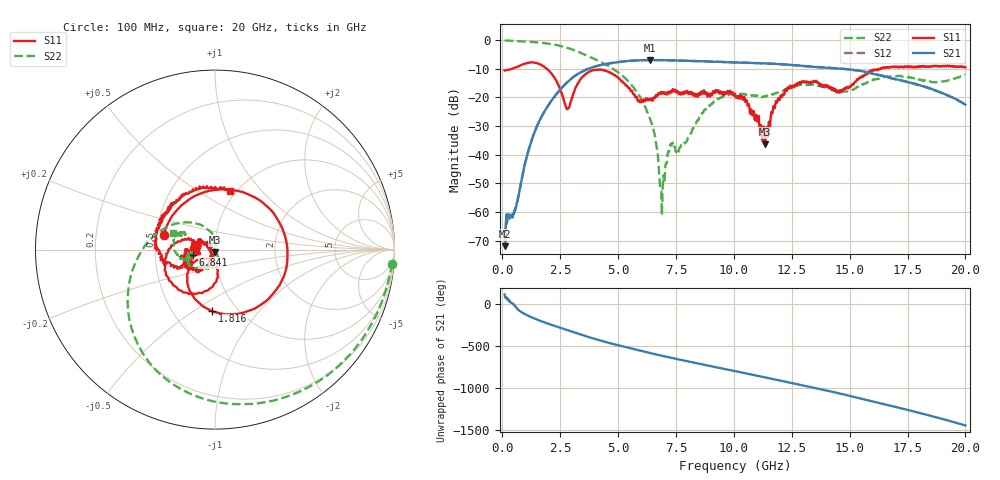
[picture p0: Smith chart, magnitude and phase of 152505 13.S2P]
!  2-Port S-parameters saved by WinCal
! VAR MeasName=S-Parameters (CALIBRATED_DATA) read from VNA (N5230C)
! VAR MeasDate=4/10/2015 9:29:35 AM
! VAR NAME=152505 13
! VAR FILENAME=152505 13.S2P
! VAR DATE=4/10/2015 9:29:35 AM
! VAR PHYS_PORTS=1,2
# Hz S DB R 50
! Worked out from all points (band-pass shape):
!   801 points, 100 MHz to 20 GHz, reference 50 ohm
!   highest |S21| = -6.92 dB at 6.393 GHz (marker M1); lowest = -71.9 dB at 124.9 MHz (marker M2)
!   |S21| within 3 dB of the highest: 3.733 GHz to 14.57 GHz (10.84 GHz wide, 118 % of centre)
!   lowest |S11| = -36.4 dB at 11.34 GHz (marker M3), VSWR 1.03, Z = 49.8 - j1.51 ohm
!   |S11| at or under -10 dB: start of sweep to 413.4 MHz; 1.927 GHz to 16.32 GHz (14.39 GHz wide, 158 % of centre)
!   |S22| runs from -61.1 to -0.1 dB; largest |S21 - S12| = 0.0063
!   S11 on the Smith chart (normalised r, x): 100 MHz: 0.55, +0.10; 1.816 GHz: 0.77, -0.60; 6.841 GHz: 0.78, -0.05; 20 GHz: 0.94, +0.69
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1e8  -10.57 164.5  -67.38 110.1  -70.23 114.6  -0.08 -4.6
1.24875e8  -10.54 160.5  -71.92 74.5  -68.42 97.4  -0.10 -5.5
6.4725e8  -9.29 77.1  -56.43 -58.5  -56.48 -58.9  -0.31 -26.3
1.095e9  -7.94 5.0  -39.47 -139.7  -39.52 -139.5  -0.50 -44.3
1.816375e9  -9.27 -92.6  -24.94 138.8  -24.94 138.9  -1.02 -74.2
2.811375e9  -23.99 -118.8  -14.63 46.1  -14.64 46.4  -2.65 -118.3
3.43325e9  -13.11 -98.1  -11.03 -10.9  -11.00 -10.6  -4.56 -145.0
4.701875e9  -11.53 -175.9  -8.02 -112.6  -8.00 -112.4  -9.54 163.8
5.5725e9  -17.67 156.1  -7.16 -173.5  -7.14 -173.7  -15.50 122.3
6.393375e9  -20.97 -167.2  -6.92 132.3  -6.93 132.3  -27.70 85.4
6.741625e9  -18.51 -168.6  -6.95 110.5  -6.93 110.2  -42.78 82.0
6.841125e9  -18.04 -166.6  -6.95 104.3  -6.97 104.0  -52.24 142.4
7.264e9  -17.75 -173.8  -7.04 78.8  -7.03 78.8  -36.29 -130.2
8.582375e9  -18.21 173.1  -7.35 1.6  -7.30 1.5  -26.42 -67.9
1.005e10  -18.74 163.2  -7.74 -81.9  -7.77 -82.1  -18.99 -115.7
1.13435e10  -36.35 -96.2  -8.08 -156.0  -8.10 -155.8  -19.47 -130.5
1.231362e10  -16.92 -128.7  -8.53 147.4  -8.51 146.9  -16.78 -134.3
1.338325e10  -14.67 -164.7  -9.27 84.2  -9.20 84.3  -15.45 -158.8
1.477625e10  -16.92 -163.0  -10.03 -1.5  -10.01 -1.9  -17.88 -168.0
1.669162e10  -9.54 171.6  -13.00 -129.6  -13.06 -130.8  -12.72 176.4
1.835825e10  -9.35 129.0  -16.46 115.8  -16.61 115.8  -14.13 151.4
2e10  -9.49 75.4  -22.49 -8.9  -22.53 -8.4  -12.04 158.4
